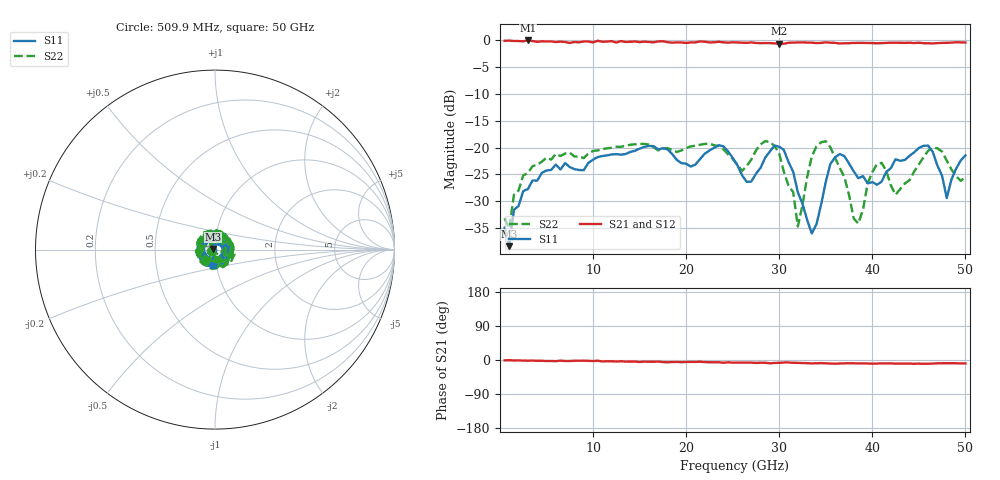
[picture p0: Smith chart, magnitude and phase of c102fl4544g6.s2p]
! 8/2/2019 3:18:19 PM
! Z:\MATT MILLER ENGINEERING\C102FL4544G6.S2P
! CHANNEL.1
! TR.MEASUREMENT
! CORRECTED.DATA
# GHZ S RI R 50.0
! FREQ.GHZ  S11RE  S11IM  S21RE  S21IM  S12RE  S12IM  S22RE  S22IM
!; PortSelection: Port_12
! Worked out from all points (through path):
!   100 points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, 509.9 MHz to 50 GHz, reference 50 ohm
!   highest |S21| = -0.02 dB at 3.009 GHz (marker M1); lowest = -0.6 dB at 30 GHz (marker M2)
!   group delay of S21, straight-line fit = 517 fs
!   lowest |S11| = -38.4 dB at 1.01 GHz (marker M3), VSWR 1.02, Z = 48.9 + j0.308 ohm
!   |S11| at or under -10 dB: start of sweep to end of sweep
!   |S22| runs from -35.1 to -18.8 dB; largest |S21 - S12| = 0.018
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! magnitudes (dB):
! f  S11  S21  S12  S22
! 509.9 MHz  -35.0  -0.1  -0.1  -33.2
! 1.01 GHz  -38.4  0.0  -0.1  -35.1
! 1.51 GHz  -31.6  -0.1  -0.1  -28.8
! 3.009 GHz  -27.7  0.0  -0.1  -24.7
! 9.008 GHz  -24.2  -0.2  -0.2  -22.0
! 17.51 GHz  -20.1  -0.2  -0.3  -20.1
! 20.51 GHz  -23.6  -0.4  -0.4  -19.8
! 23.51 GHz  -19.6  -0.3  -0.2  -19.7
! 25.5 GHz  -23.3  -0.4  -0.5  -23.2
! 27 GHz  -26.4  -0.4  -0.4  -22.3
! 30 GHz  -19.8  -0.6  -0.7  -21.1
! 31.5 GHz  -24.5  -0.4  -0.4  -28.3
! 32 GHz  -28.3  -0.4  -0.4  -34.7
! 33.5 GHz  -36.0  -0.4  -0.4  -21.7
! 35 GHz  -26.4  -0.4  -0.5  -18.8
! 36 GHz  -21.8  -0.5  -0.5  -21.9
! 38.5 GHz  -25.7  -0.5  -0.4  -34.2
! 40.5 GHz  -26.9  -0.5  -0.5  -23.1
! 42 GHz  -23.8  -0.4  -0.5  -27.1
! 46 GHz  -19.7  -0.6  -0.6  -20.6
! 48 GHz  -29.4  -0.5  -0.4  -22.4
! 50 GHz  -21.5  -0.4  -0.5  -25.5
